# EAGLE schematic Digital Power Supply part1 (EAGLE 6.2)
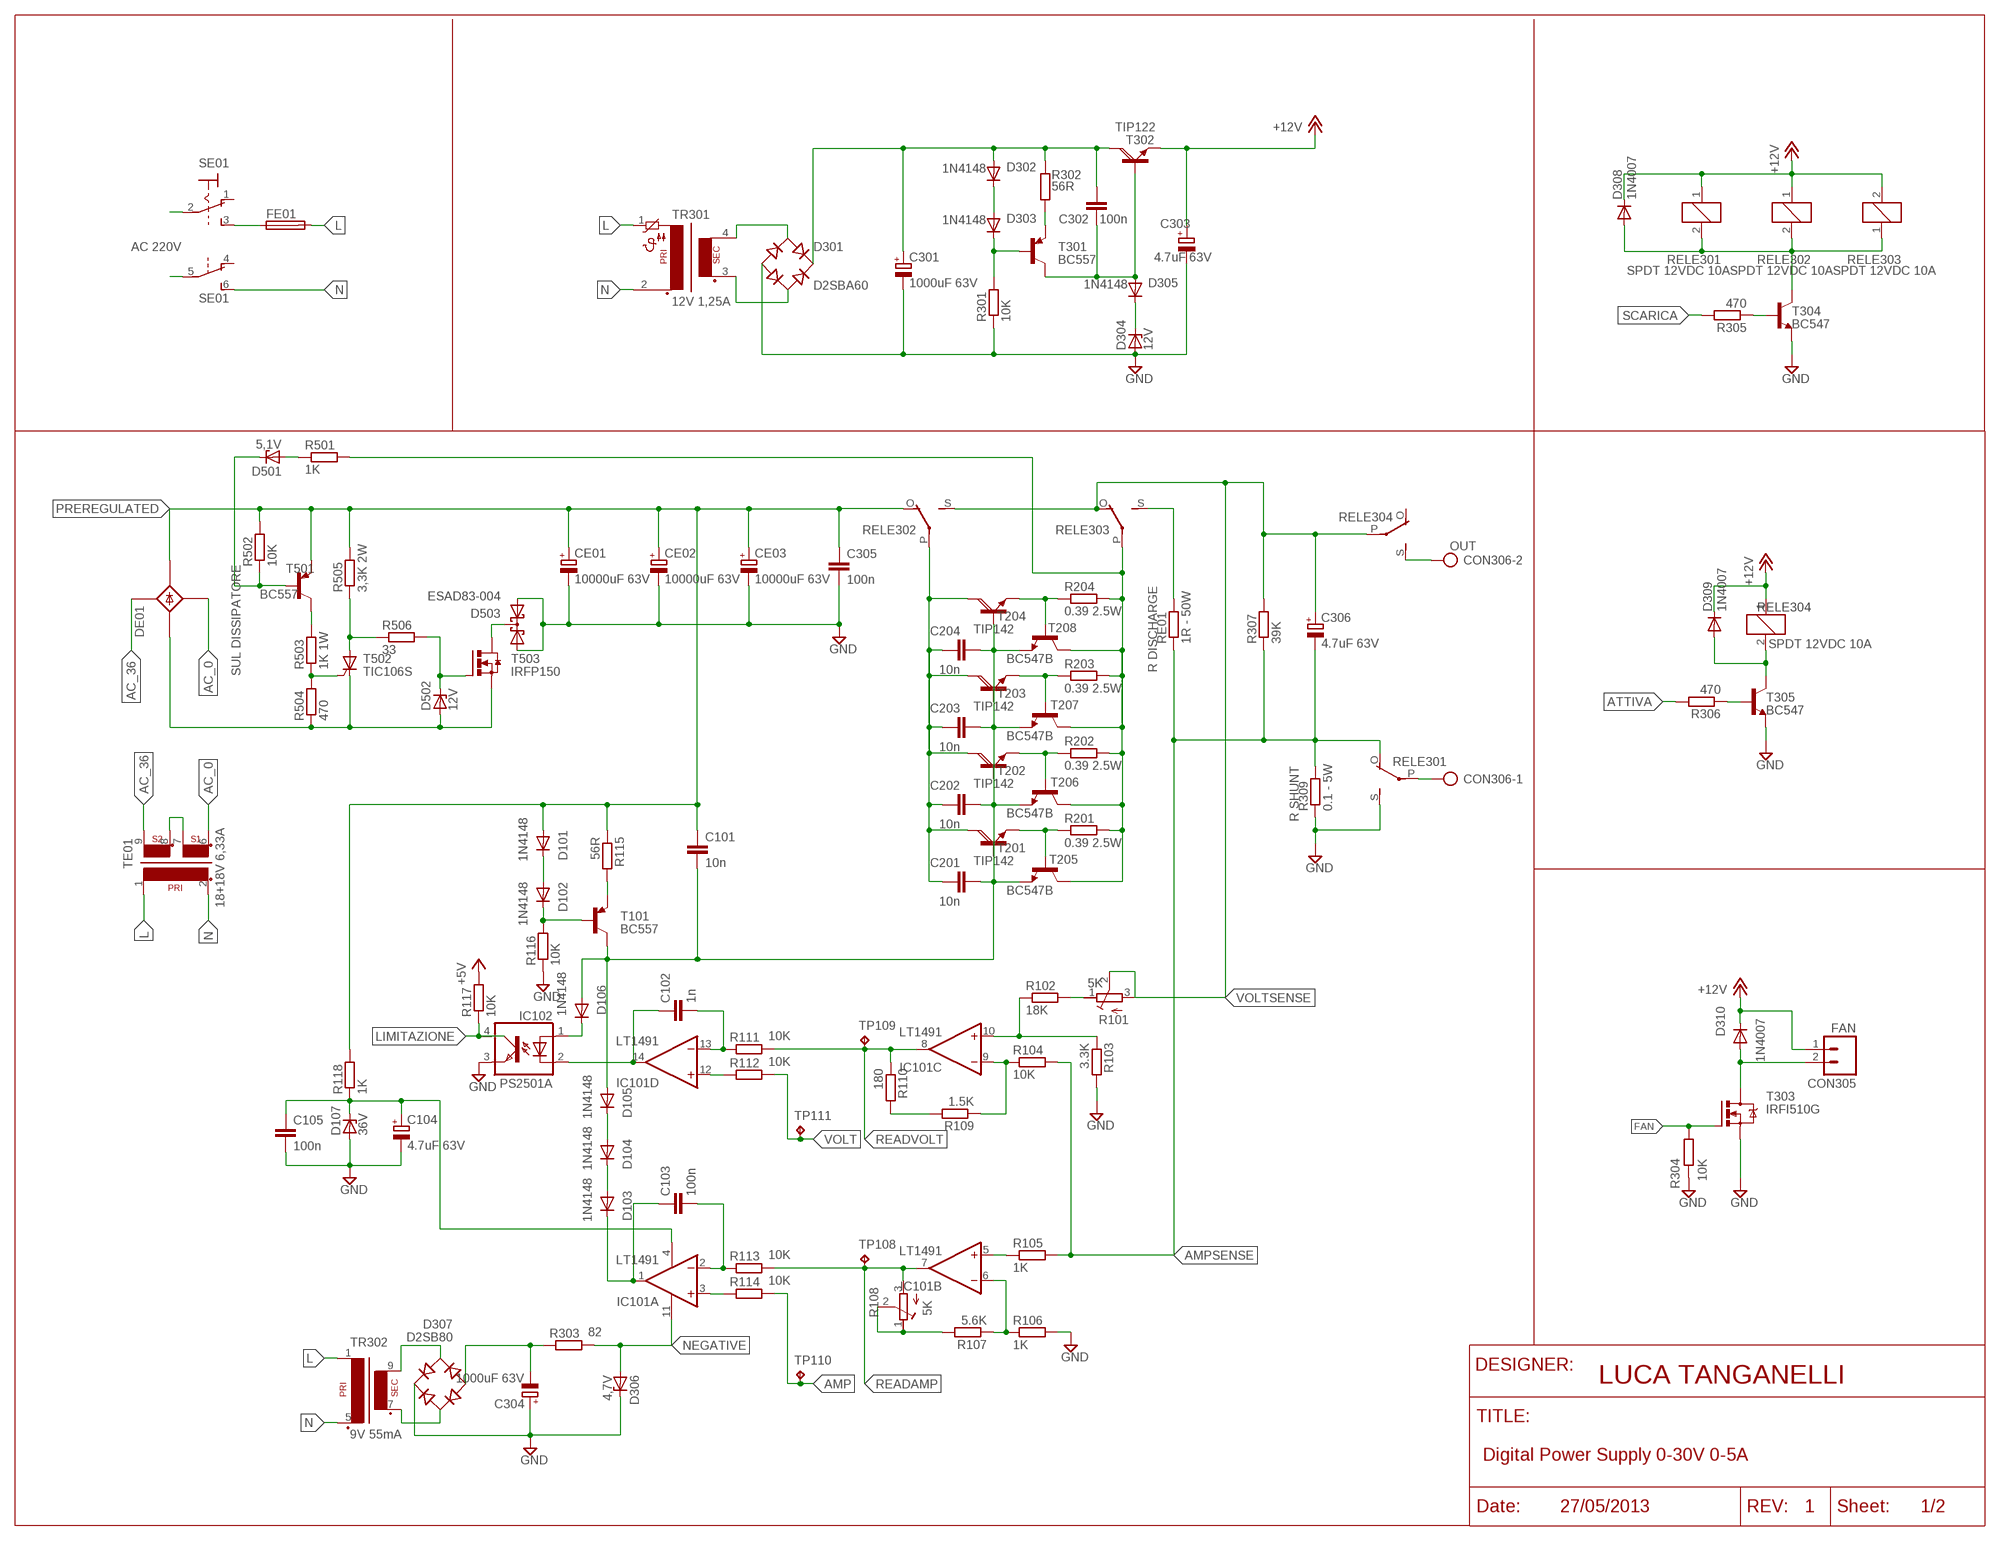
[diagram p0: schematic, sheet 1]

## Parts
C101  10n  C-EU050-024X044  [C050-024X044]
C102  1n  C-EU050-024X044  [C050-024X044]
C103  100n  C-EU050-024X044  [C050-024X044]
C104  4.7uF 63V  CPOL-EUE2.5-5  [E2,5-5]
C105  100n  C-EU050-024X044  [C050-024X044]
C201  10n  C-EU050-024X044  [C050-024X044]
C202  10n  C-EU050-024X044  [C050-024X044]
C203  10n  C-EU050-024X044  [C050-024X044]
C204  10n  C-EU050-024X044  [C050-024X044]
C301  1000uF 63V  CPOL-EUE7.5-16  [E7,5-16]
C302  100n  C-EU050-024X044  [C050-024X044]
C303  4.7uF 63V  CPOL-EUE2.5-5  [E2,5-5]
C304  1000uF 63V  CPOL-EUE7.5-16  [E7,5-16]
C305  100n  C-EU050-024X044  [C050-024X044]
C306  4.7uF 63V  CPOL-EUE2.5-5  [E2,5-5]
CE01  10000uF 63V  CPOL-EUE10-35  [EB35D]
CE02  10000uF 63V  CPOL-EUE10-35  [EB35D]
CE03  10000uF 63V  CPOL-EUE10-35  [EB35D]
CON305  FAN  M02  [02P]
CON306  OUT  AK500/2  [AK500/2]
D101  1N4148  1N4148DO35-7  [DO35-7]
D102  1N4148  1N4148DO35-7  [DO35-7]
D103  1N4148  1N4148DO35-10  [DO35-10]
D104  1N4148  1N4148DO35-10  [DO35-10]
D105  1N4148  1N4148DO35-10  [DO35-10]
D106  1N4148  1N4148DO35-10  [DO35-10]
D107  36V  1N4728  [DO41Z10]
D301  D2SBA60  RECTIFIER-GBU4S  [GBU4S]
D302  1N4148  1N4148DO35-7  [DO35-7]
D303  1N4148  1N4148DO35-7  [DO35-7]
D304  12V  BZX85  [DO41Z10]
D305  1N4148  1N4148DO35-7  [DO35-7]
D306  4,7V  1N4728  [DO41Z10]
D307  D2SB80  RECTIFIER-GBU4S  [GBU4S]
D308  1N4007  1N4004  [DO41-10]
D309  1N4007  1N4004  [DO41-10]
D310  1N4007  1N4004  [DO41-10]
D501  5,1V  ZENER-DIODEDO35Z10  [DO35Z10]
D502  12V  ZENER-DIODEDO35Z10  [DO35Z10]
D503  ESAD83-004  ESAD83-004TO247BV  [TO247BV]
DE01  SUL DISSIPATORE  B25A-  [B25A-]
FE01  KS17  [KS17]
IC101  LT1491  TL084P  [DIL14]
IC102  PS2501A  TIL191  [DIL04]
R101  5K  R-TRIMMT93YA  [RTRIMT93YA]
R102  18K  R-EU_0207/10  [0207/10]
R103  3.3K  R-EU_0207/10  [0207/10]
R104  10K  R-EU_0207/12  [0207/12]
R105  1K  R-EU_0207/10  [0207/10]
R106  1K  R-EU_0207/10  [0207/10]
R107  5.6K  R-EU_0207/10  [0207/10]
R108  5K  R-TRIMMT93YA  [RTRIMT93YA]
R109  1.5K  R-EU_0207/10  [0207/10]
R110  180  R-EU_0207/10  [0207/10]
R111  10K  R-EU_0207/12  [0207/12]
R112  10K  R-EU_0207/10  [0207/10]
R113  10K  R-EU_0207/10  [0207/10]
R114  10K  R-EU_0207/10  [0207/10]
R115  56R  R-EU_0207/10  [0207/10]
R116  10K  R-EU_0207/10  [0207/10]
R117  10K  R-EU_0207/10  [0207/10]
R118  1K  R-EU_0309/12  [0309/12]
R201  0.39 2.5W  R-EU_0411/15  [0411/15]
R202  0.39 2.5W  R-EU_0411/15  [0411/15]
R203  0.39 2.5W  R-EU_0411/15  [0411/15]
R204  0.39 2.5W  R-EU_0411/15  [0411/15]
R301  10K  R-EU_0207/10  [0207/10]
R302  56R  R-EU_0207/10  [0207/10]
R303  82  R-EU_0207/10  [0207/10]
R304  10K  R-EU_0207/10  [0207/10]
R305  470  R-EU_0207/10  [0207/10]
R306  470  R-EU_0207/10  [0207/10]
R307  39K  R-EU_0207/10  [0207/10]
R309  0.1 - 5W  R-EU_0921/26  [0921/26]
R501  1K  R-EU_0207/26  [0207/26]
R502  10K  R-EU_0207/10  [0207/10]
R503  1K 1W  R-EU_0921/26  [0921/26]
R504  470  R-EU_0207/10  [0207/10]
R505  3,3K 2W  R-EU_0921/26  [0921/26]
R506  33  R-EU_0207/10  [0207/10]
RE01  1R - 50W  R-EU_0921/26  [0921/26]
RELE301  SPDT 12VDC 10A  ZF112  [ZF112]
RELE302  SPDT 12VDC 10A  ZF112  [ZF112]
RELE303  SPDT 12VDC 10A  ZF112  [ZF112]
RELE304  SPDT 12VDC 10A  ZF112  [ZF112]
SE01  320-938  [320-938]
T101  BC557  [TO92-EBC]
T201  TIP142  [TO247BV]
T202  TIP142  [TO247BV]
T203  TIP142  [TO247BV]
T204  TIP142  [TO247BV]
T205  BC547B  BC547B-NPN-TO92-CBE  [TO92-CBE]
T206  BC547B  BC547B-NPN-TO92-CBE  [TO92-CBE]
T207  BC547B  BC547B-NPN-TO92-CBE  [TO92-CBE]
T208  BC547B  BC547B-NPN-TO92-CBE  [TO92-CBE]
T301  BC557  [TO92-EBC]
T302  TIP122  [TO220AV]
T303  IRFI510G  IRF520  [TO220BV]
T304  BC547  BC547-NPN-TO92-CBE  [TO92-CBE]
T305  BC547  BC547-NPN-TO92-CBE  [TO92-CBE]
T501  BC557  BC557A-PNP-TO92-CBE  [TO92-CBE]
T502  TIC106S  [TIC106S]
T503  IRFP150  IRFP240  [TO247BV]
TE01  18+18V 6,33A  TOROIDE  [TOROIDE1P2S]
TP108  TP  [TP1]
TP109  TP  [TP1]
TP110  TP  [TP1]
TP111  TP  [TP1]
TR301  12V 1,25A  PT04,5-1  [PT04,5-1]
TR302  9V 55mA  VR11  [VR11]

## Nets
36V: C104.+ C105.1 D107.C IC101.4(P:V+) R118.1
+5V: R117.2
+12V: C303.+ CON305.1 D308.C D309.C D310.C RELE301.1 RELE302.1 RELE303.2 RELE304.1 T302.E
AC_0: D301.AC2 DE01.AC2-(AC2) TE01.6 TR301.3
AC_18: D301.AC1 TE01.7 TE01.8 TR301.4
AC_36: DE01.AC1-(AC1) TE01.9
AMP: R114.2 TP110.P$1(TP)
AMPSENSE: C306.- R104.2 R105.2 R307.1 R309.P$2 RE01.P$1 RELE301.O(2:O)
ATTIVA: R306.2
DISCHARGE: RE01.P$2 RELE303.S(2:S)
FAN: R304.1 T303.G
GND: C104.- C105.2 C301.- C303.- C304.+ C305.2 CE01.- CE02.- CE03.- D107.A D301.- D304.A D306.C D307.+ D503.B(A1) D503.E(A2) IC102.3(EMIT) R103.2 R106.2 R116.1 R301.1 R304.2 R309.P$1 RELE301.S(2:S) T303.S T304.E T305.E
L: FE01.2 TE01.1 TR301.1 TR302.1
LIMITAZIONE: IC102.4(COL) R117.1
N: SE01.6(B:S) TE01.2 TR301.2 TR302.5(P2)
N$1: IC101.5(B:+IN) R105.1
N$2: IC101.6(B:-IN) R106.1 R107.1
N$3: IC101.10(C:+IN) R102.1 R103.1
N$4: IC101.9(C:-IN) R104.1 R109.1
N$5: C102.2 IC101.13(D:-IN) R111.1
N$6: IC101.12(D:+IN) R112.1
N$7: C103.2 IC101.2(A:-IN) R113.1
N$8: IC101.3(A:+IN) R114.1
N$9: R107.2 R108.1(A) R108.2(S)
N$12: CON306.1 RELE301.P(2:P)
N$13: R101.1(A) R102.2
N$14: R109.2 R110.2
N$15: D304.C D305.C
N$17: C102.1 IC101.14(D:OUT) IC102.2(C)
N$18: C103.1 D103.C IC101.1(A:OUT)
N$19: SE01.2(1:P)
N$20: R115.2 T101.E
N$21: D101.C D102.A
N$22: D102.C R116.2 T101.B
N$24: D307.AC2 TR302.9(S4)
N$25: SE01.5(B:P)
N$26: D307.AC1 TR302.7(S3)
N$27: CON306.2 RELE304.S(2:S)
N$28: C304.- D307.- R303.1
N$29: D503.C T503.C(D)
N$31: FE01.1 SE01.3(1:S)
N$38: R204.1 T204.E T208.B
N$39: R203.1 T203.E T207.B
N$40: R202.1 T202.E T206.B
N$41: R201.1 T201.E T205.B
N$43: C302.1 D305.A T301.C T302.B
N$44: C301.+ C302.2 D301.+ D302.A R302.1 T302.C
N$45: D106.C IC102.1(A)
N$46: D302.C D303.A
N$47: D303.C R301.2 T301.B
N$49: R302.2 T301.E
N$52: D103.A D104.C
N$53: D502.A DE01.-1(-) R504.1 T502.C T503.E(S)
N$55: R305.1 T304.B
N$57: D308.A RELE301.2 RELE302.2 RELE303.1 T304.C
N$58: D502.C R506.2 T503.B(G)
N$59: R503.P$1 R504.2 T502.G
N$62: R306.1 T305.B
N$64: D309.A RELE304.2 T305.C
N$71: R505.P$1 R506.1 T502.A
N$73: R503.P$2 T501.C
N$74: D501.C R502.1 T501.B
N$75: D501.A R501.1
N$76: D104.A D105.C
N$94: CON305.2 D310.A T303.D
NEGATIVE: D306.A IC101.11(P:V-) R303.2
POWER_IN: C201.1 C202.1 C203.1 C204.1 RELE302.P(2:P) T201.C T202.C T203.C T204.C
POWER_OUT: R201.2 R202.2 R203.2 R204.2 R501.2 RELE303.P(2:P) T205.C T206.C T207.C T208.C
PREREGULATED: C101.1 C305.1 CE01.+ CE02.+ CE03.+ D101.A DE01.+1(+) R115.1 R118.2 R502.2 R505.P$2 RELE302.O(2:O) T501.E
READAMP: IC101.7(B:OUT) R108.3(E) R113.2 TP108.P$1(TP)
READVOLT: IC101.8(C:OUT) R110.1 R111.2 TP109.P$1(TP)
REG: C101.2 C201.2 C202.2 C203.2 C204.2 D105.A D106.A T101.C T201.B T202.B T203.B T204.B T205.E T206.E T207.E T208.E
SCARICA: R305.2
VOLT: R112.2 TP111.P$1(TP)
VOLTSENSE: C306.+ R101.2(S) R101.3(E) R307.2 RELE302.S(2:S) RELE303.O(2:O) RELE304.P(2:P)
Unconnected: DE01.+ DE01.- DE01.AC1 DE01.AC2 RELE304.O(2:O) SE01.1(1:O) SE01.4(B:O)

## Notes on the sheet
- AC 220V
- R DISCHARGE
- R SHUNT
- LUCA TANGANELLI
- Digital Power Supply 0-30V 0-5A
- 27/05/2013 | 1 | 1/2

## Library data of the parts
C101-C103 C105 C201-C204 C302 C305 = #-rcl:C-EU: CAPACITOR, European symbol
C104 C301 C303 C304 C306 CE01-CE03 = #-rcl:CPOL-EU: POLARIZED CAPACITOR, European symbol
CON305 = #-con-amp-quick:M02: AMP QUICK CONNECTOR; OC_FARNELL: unknown; OC_NEWARK: unknown
CON306 = #-con-ptr500:AK500/2: CONNECTOR; OC_FARNELL: unknown; OC_NEWARK: unknown
D101-D106 D302 D303 D305 = #-diode:1N4148: DIODE
D107 D306 = #-diode:1N4728: Z DIODE
D301 D307 = #-rectifier:RECTIFIER-: Rectifier
D304 = #-diode:BZX85: Z DIODE
D308-D310 = #-diode:1N4004: DIODE
D501 D502 = #-diode:ZENER-DIODE: Z-Diode
D503 = #-diode:ESAD83-004
DE01 = rectifier:B25A-: RECTIFIER 25-A bridge
FE01 = fuse:KS17: FUSE HOLDER; OC_FARNELL: unknown; OC_NEWARK: unknown
IC101 = #-linear:TL084: OP AMP
IC102 = #-optocoupler:TIL191: TEXAS INSTRUMENTS OPTO COUPLER; OC_FARNELL: 1683363; OC_NEWARK: unknown
R101 R108 = #-rcl:R-TRIMM: Trimm resistor
R102-R107 R109-R118 R201-R204 R301-R307 R309 R501-R506 RE01 = #-rcl:R-EU_: RESISTOR, European symbol
RELE301-RELE304 = relay:ZF112: RELAY 1 x switch; OC_FARNELL: unknown; OC_NEWARK: unknown
SE01 = switch:320-938: TOGGLE SWITCH distributor RS Components
T101 T301 = #-transistor-pnp:BC557*: PNP Transistror
T201-T204 = #-transistor-power:TIP142: NPN DARLINGTON TRANSISTOR
T205-T208 T304 T305 = #-transistor:*-NPN-: NPN Transistror BF959 corrected 2008.03.06
T302 = #-transistor-power:TIP122
T303 = #-transistor-power:IRF520: HEXFET Power MOSFET
T501 = #-transistor:*-PNP-: PNP Transistror
T502 = triac:TIC106S: THYRISTOR
T503 = #-transistor-power:IRFP240: HEXFET Power MosFet Source: http://www.irf.com/
TE01 = #-trafo:TOROIDE: Trasformatore Toroidale
TP108-TP111 = #-testpad:TP: Test pad
TR301 = #-trafo:PT04,5-1: TRANSFORMER 1 primary winding, temp. protection fuse, 1 secondary winding/ mounting hole BLOCK
TR302 = #-trafo:VR11: TRANSFORMER 1 primary winding, 1 secondary winding BLOCK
